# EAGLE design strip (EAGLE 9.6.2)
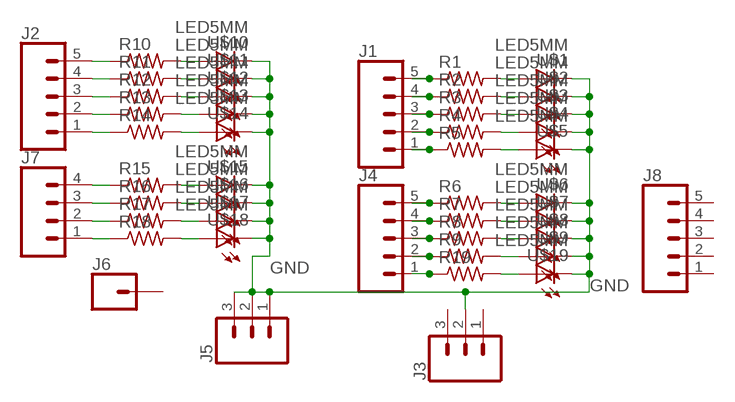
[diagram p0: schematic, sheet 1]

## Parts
J1  CONN_05PTH_LONGPADS  [1X05_LONGPADS]
J2  CONN_05PTH_LONGPADS  [1X05_LONGPADS]
J3  CONN_03LONGPADS  [1X03_LONGPADS]
J4  CONN_05PTH_LONGPADS  [1X05_LONGPADS]
J5  CONN_03LONGPADS  [1X03_LONGPADS]
J6  CONN_01PTH_LONGPAD  [1X01_LONGPAD]
J7  CONN_04LONGPADS  [1X04_LONGPADS]
J8  CONN_05PTH_LONGPADS  [1X05_LONGPADS]
R1  RES-US1206FAB  [R1206FAB]
R2  RES-US1206FAB  [R1206FAB]
R3  RES-US1206FAB  [R1206FAB]
R4  RES-US1206FAB  [R1206FAB]
R5  RES-US1206FAB  [R1206FAB]
R6  RES-US1206FAB  [R1206FAB]
R7  RES-US1206FAB  [R1206FAB]
R8  RES-US1206FAB  [R1206FAB]
R9  RES-US1206FAB  [R1206FAB]
R10  RES-US1206FAB  [R1206FAB]
R11  RES-US1206FAB  [R1206FAB]
R12  RES-US1206FAB  [R1206FAB]
R13  RES-US1206FAB  [R1206FAB]
R14  RES-US1206FAB  [R1206FAB]
R15  RES-US1206FAB  [R1206FAB]
R16  RES-US1206FAB  [R1206FAB]
R17  RES-US1206FAB  [R1206FAB]
R18  RES-US1206FAB  [R1206FAB]
R19  RES-US1206FAB  [R1206FAB]
U$1  LED5MM  [5MM]
U$2  LED5MM  [5MM]
U$3  LED5MM  [5MM]
U$4  LED5MM  [5MM]
U$5  LED5MM  [5MM]
U$6  LED5MM  [5MM]
U$7  LED5MM  [5MM]
U$8  LED5MM  [5MM]
U$9  LED5MM  [5MM]
U$10  LED5MM  [5MM]
U$11  LED5MM  [5MM]
U$12  LED5MM  [5MM]
U$13  LED5MM  [5MM]
U$14  LED5MM  [5MM]
U$15  LED5MM  [5MM]
U$16  LED5MM  [5MM]
U$17  LED5MM  [5MM]
U$18  LED5MM  [5MM]
U$19  LED5MM  [5MM]

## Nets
GND: J3.2 J5.1 J5.2 J5.3 U$1.OUT(C) U$2.OUT(C) U$3.OUT(C) U$4.OUT(C) U$5.OUT(C) U$6.OUT(C) U$7.OUT(C) U$8.OUT(C) U$9.OUT(C) U$10.OUT(C) U$11.OUT(C) U$12.OUT(C) U$13.OUT(C) U$14.OUT(C) U$15.OUT(C) U$16.OUT(C) U$17.OUT(C) U$18.OUT(C) U$19.OUT(C)
N$1: J1.5 R1.1
N$2: J1.4 R2.1
N$3: J1.3 R3.1
N$4: J1.2 R4.1
N$5: J1.1 R5.1
N$6: J4.5 R6.1
N$7: J4.4 R7.1
N$8: J4.3 R8.1
N$9: J4.2 R9.1
N$10: J2.5 R10.1
N$11: J2.4 R11.1
N$12: J2.3 R12.1
N$13: J2.2 R13.1
N$14: J2.1 R14.1
N$15: J7.4 R15.1
N$16: J7.1 R18.1
N$17: J7.2 R17.1
N$18: J7.3 R16.1
N$19: R1.2 U$1.IN(A)
N$20: R2.2 U$2.IN(A)
N$21: R3.2 U$3.IN(A)
N$22: R4.2 U$4.IN(A)
N$23: R5.2 U$5.IN(A)
N$24: R6.2 U$6.IN(A)
N$25: R7.2 U$7.IN(A)
N$26: R8.2 U$8.IN(A)
N$27: R9.2 U$9.IN(A)
N$28: R10.2 U$10.IN(A)
N$29: R11.2 U$11.IN(A)
N$30: R12.2 U$12.IN(A)
N$31: R13.2 U$13.IN(A)
N$32: R14.2 U$14.IN(A)
N$33: R15.2 U$15.IN(A)
N$34: R16.2 U$16.IN(A)
N$35: R17.2 U$17.IN(A)
N$36: R18.2 U$18.IN(A)
N$37: R19.2 U$19.IN(A)
N$38: J4.1 R19.1
Unconnected: J3.1 J3.3 J6.1 J8.1 J8.2 J8.3 J8.4 J8.5

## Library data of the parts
J1 J2 J4 J8 = SparkFun-Connectors:CONN_05: Multi connection point. Often used as Generic Header-pin footprint for 0.1 inch spaced/style header connections On any of the 0.1 inch spaced packages, you can populate with these: Break Away Headers - Straight (PRT-00116) Break Away Male Headers - Right Angle (PRT-00553) Female Headers (PRT-00115)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
J3 J5 = SparkFun-Connectors:CONN_03: Multi connection point. Often used as Generic Header-pin footprint for 0.1 inch spaced/style header connections On any of the 0.1 inch spaced packages, you can populate with these: Break Away Headers - Straight (PRT-00116) Break Away Male Headers - Right Angle (PRT-00553) Female Headers (PRT-00115)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
J6 = SparkFun-Connectors:CONN_01: Single connection point. Often used as Generic Header-pin footprint for 0.1 inch spaced/style header connections
J7 = SparkFun-Connectors:CONN_04: Multi connection point. Often used as Generic Header-pin footprint for 0.1 inch spaced/style header connections On any of the 0.1 inch spaced packages, you can populate with these: Break Away Headers - Straight (PRT-00116) Break Away Male Headers - Right Angle (PRT-00553) Female Headers (PRT-00115)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; PROD_ID: CONN-09696
R1-R19 = fab:RES-US: Resistor (US Symbol)
U$1-U$19 = fab:LED: LED

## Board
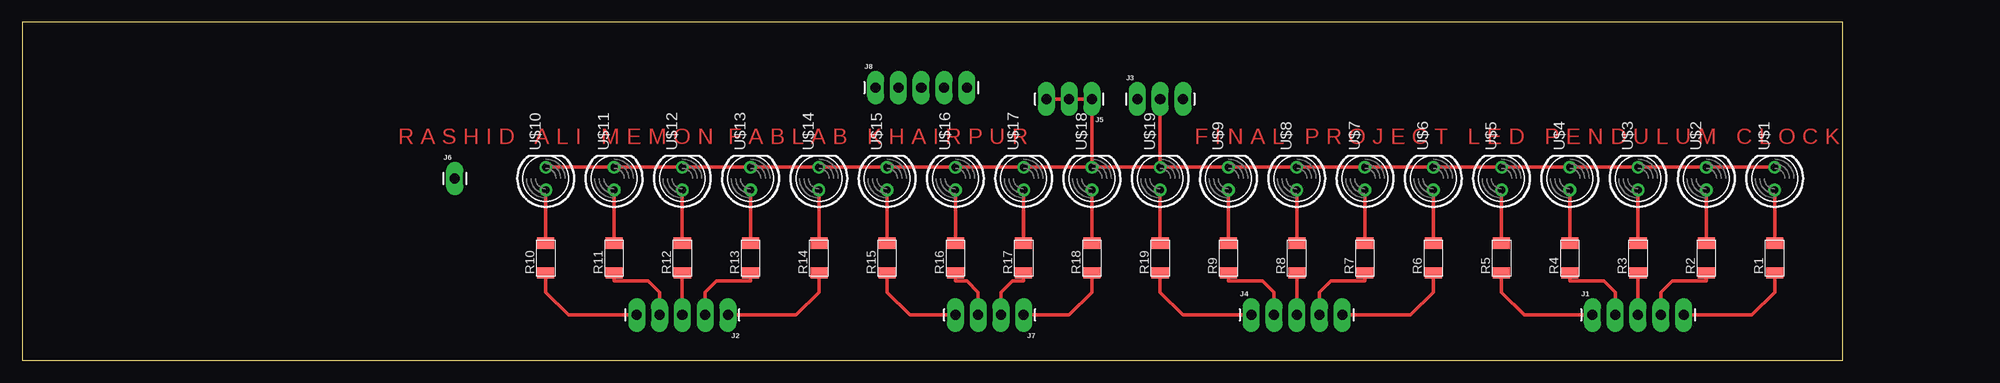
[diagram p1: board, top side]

Size 203.18 x 37.77 mm. Coordinates in mm from the lower left corner, seen from the top.
Outline: 0,0 203.18,0 203.18,37.77 0,37.77 0,0
Copper layers (1*16): Top 0.035mm / dielectric 1.5mm / Bottom 0.035mm
Design rules "default": minimum track width 6mil, minimum drill 0.35mm, track to track 6mil, track to pad 6mil, pad to pad 6mil, via to via 6mil, smd to smd 6mil, copper to edge 40mil, drill to drill 6mil, minimum pad ring 10mil, minimum via ring 8mil, stop-mask expansion 4mil, vias tented up to drill 0mil, thermal gap 10mil

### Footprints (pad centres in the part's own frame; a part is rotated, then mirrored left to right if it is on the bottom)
1X05_LONGPADS = drill 1.118 pad 1.88 long: 1 0,0; 2 2.54,0; 3 5.08,0; 4 7.62,0; 5 10.16,0
1X03_LONGPADS = drill 1.118 pad 1.88 long: 1 0,0; 2 2.54,0; 3 5.08,0
1X01_LONGPAD = drill 1.118 pad 1.88 long: 1 0,0
1X04_LONGPADS = drill 1.118 pad 1.88 long: 1 0,0; 2 2.54,0; 3 5.08,0; 4 7.62,0
R1206FAB = smd 1.27 x 1.905: 1 -1.651,0; 2 1.651,0
5MM = drill 0.813 pad 1.422: IN -1.27,0; OUT 1.27,0

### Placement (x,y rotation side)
J1  175.26,5.08 0 top
J2  78.74,5.08 180 top
J3  124.46,29.21 0 top
J4  137.16,5.08 0 top
J5  119.38,29.21 180 top
J6  48.26,20.32 0 top
J7  111.76,5.08 180 top
J8  95.25,30.48 0 top
R1  195.58,11.43 90 top
R2  187.96,11.43 90 top
R3  180.34,11.43 90 top
R4  172.72,11.43 90 top
R5  165.1,11.43 90 top
R6  157.48,11.43 90 top
R7  149.86,11.43 90 top
R8  142.24,11.43 90 top
R9  134.62,11.43 90 top
R10  58.42,11.43 90 top
R11  66.04,11.43 90 top
R12  73.66,11.43 90 top
R13  81.28,11.43 90 top
R14  88.9,11.43 90 top
R15  96.52,11.43 90 top
R16  104.14,11.43 90 top
R17  111.76,11.43 90 top
R18  119.38,11.43 90 top
R19  127,11.43 90 top
U$1  195.58,20.32 90 top
U$2  187.96,20.32 90 top
U$3  180.34,20.32 90 top
U$4  172.72,20.32 90 top
U$5  165.1,20.32 90 top
U$6  157.48,20.32 90 top
U$7  149.86,20.32 90 top
U$8  142.24,20.32 90 top
U$9  134.62,20.32 90 top
U$10  58.42,20.32 90 top
U$11  66.04,20.32 90 top
U$12  73.66,20.32 90 top
U$13  81.28,20.32 90 top
U$14  88.9,20.32 90 top
U$15  96.52,20.32 90 top
U$16  104.14,20.32 90 top
U$17  111.76,20.32 90 top
U$18  119.38,20.32 90 top
U$19  127,20.32 90 top

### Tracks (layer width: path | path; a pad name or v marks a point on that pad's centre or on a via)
GND
  Top 0.406: U$10.OUT U$11.OUT U$12.OUT U$13.OUT U$14.OUT U$15.OUT U$16.OUT U$17.OUT U$18.OUT | U$19.OUT U$18.OUT | U$19.OUT U$9.OUT U$8.OUT U$7.OUT U$6.OUT U$5.OUT U$4.OUT U$3.OUT U$2.OUT U$1.OUT | J3.2 U$19.OUT | U$18.OUT J5.1 J5.2 J5.3
N$1
  Top 0.406: R1.1 195.58,7.62 193.04,5.08 J1.5
N$2
  Top 0.406: J1.4 182.88,7.62 184.15,8.89 187.96,8.89 R2.1
N$3
  Top 0.406: J1.3 R3.1
N$4
  Top 0.406: J1.2 177.8,7.62 176.53,8.89 172.72,8.89 R4.1
N$5
  Top 0.406: J1.1 167.64,5.08 165.1,7.62 R5.1
N$6
  Top 0.406: J4.5 154.94,5.08 157.48,7.62 R6.1
N$7
  Top 0.406: J4.4 144.78,7.62 146.05,8.89 149.86,8.89 R7.1
N$8
  Top 0.406: J4.3 R8.1
N$9
  Top 0.406: J4.2 139.7,7.62 138.43,8.89 134.62,8.89 R9.1
N$10
  Top 0.406: J2.5 60.96,5.08 58.42,7.62 R10.1
N$11
  Top 0.406: J2.4 71.12,7.62 69.85,8.89 66.04,8.89 R11.1
N$12
  Top 0.406: J2.3 R12.1
N$13
  Top 0.406: J2.2 76.2,7.62 77.47,8.89 81.28,8.89 R13.1
N$14
  Top 0.406: J2.1 86.36,5.08 88.9,7.62 R14.1
N$15
  Top 0.406: J7.4 99.06,5.08 96.52,7.62 R15.1 96.52,10.16
N$16
  Top 0.406: J7.1 116.84,5.08 119.38,7.62 R18.1
N$17
  Top 0.406: J7.2 109.22,7.62 110.49,8.89 111.76,8.89 R17.1
N$18
  Top 0.406: J7.3 106.68,7.62 105.41,8.89 104.14,8.89 R16.1
N$19
  Top 0.406: U$1.IN R1.2
N$20
  Top 0.406: U$2.IN R2.2
N$21
  Top 0.406: U$3.IN R3.2
N$22
  Top 0.406: U$4.IN R4.2
N$23
  Top 0.406: U$5.IN R5.2
N$24
  Top 0.406: U$6.IN R6.2
N$25
  Top 0.406: U$7.IN R7.2
N$26
  Top 0.406: U$8.IN R8.2
N$27
  Top 0.406: U$9.IN R9.2
N$28
  Top 0.406: U$10.IN R10.2
N$29
  Top 0.406: U$11.IN R11.2
N$30
  Top 0.406: U$12.IN R12.2
N$31
  Top 0.406: U$13.IN R13.2
N$32
  Top 0.406: U$14.IN R14.2
N$33
  Top 0.406: U$15.IN R15.2
N$34
  Top 0.406: U$16.IN R16.2
N$35
  Top 0.406: U$17.IN R17.2
N$36
  Top 0.406: U$18.IN R18.2
N$37
  Top 0.406: U$19.IN R19.2
N$38
  Top 0.406: J4.1 129.54,5.08 127,7.62 R19.1

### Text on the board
Top: R A S H I D A L I M E M O N | F A B L A B K H A I R P U R | F I N A L P R O J E C T L E D P E N D U L U M C L O C K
